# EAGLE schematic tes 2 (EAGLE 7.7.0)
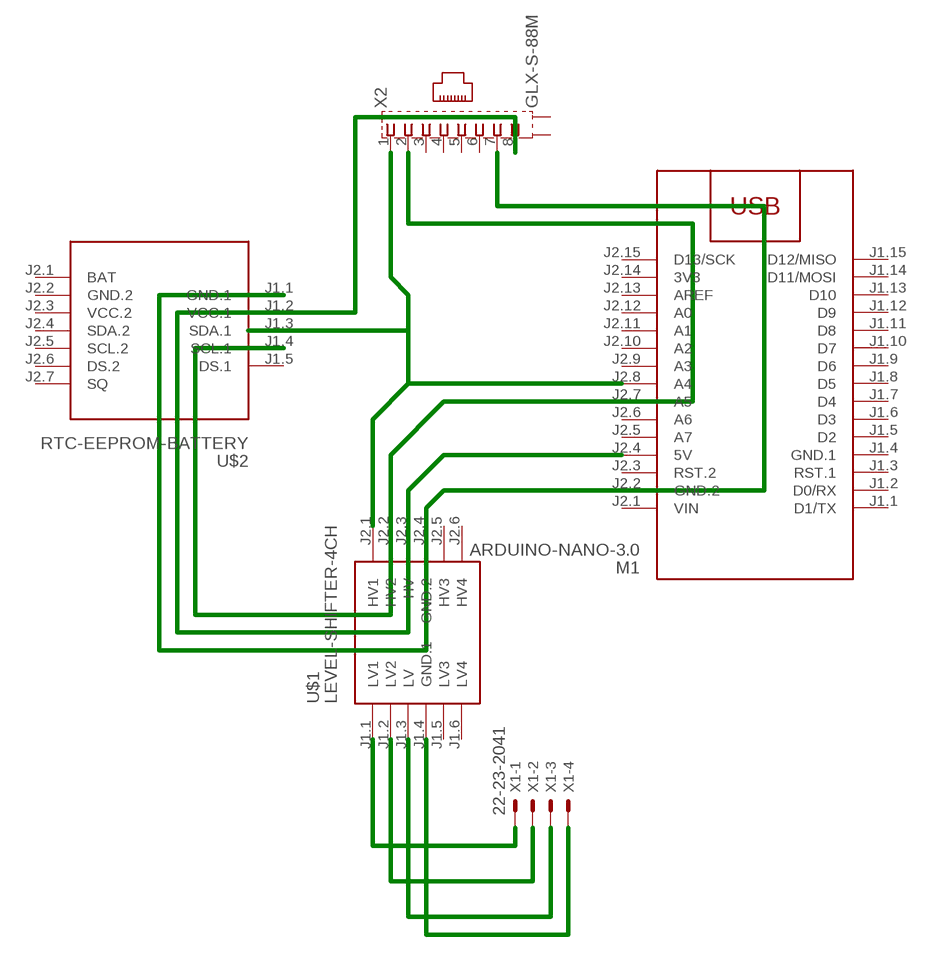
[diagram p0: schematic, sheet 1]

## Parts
M1  ARDUINO-NANO-3.0  [ARDUINO-NANO-3.0]
U$1  LEVEL-SHIFTER-4CH  [LEVEL-SHIFTER-4CH]
U$2  RTC-EEPROM-BATTERY  [RTC-EEPROM-BATTERY]
X1  22-23-2041  [22-23-2041]
X2  GLX-S-88M  [GLX-S-88M]

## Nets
N$1: M1.J2.2(GND.2) U$1.J2.4(GND.2) U$2.J1.1(GND.1) X2.7
N$2: M1.J2.4(5V) U$1.J2.3(HV) U$2.J1.2(VCC.1) X2.8
N$4: M1.J2.8(A4) U$1.J2.1(HV1) X2.1
N$5: U$1.J1.1(LV1) X1.1
N$6: U$1.J1.2(LV2) X1.2
N$7: U$1.J1.3(LV) X1.3
N$8: U$1.J1.4(GND.1) X1.4
N$9: M1.J2.7(A5) U$1.J2.2(HV2) U$2.J1.4(SCL.1) X2.2
Unconnected: M1.J1.1(D1/TX) M1.J1.2(D0/RX) M1.J1.3(RST.1) M1.J1.5(D2) M1.J1.6(D3) M1.J1.7(D4) M1.J1.8(D5) M1.J1.9(D6) M1.J1.10(D7) M1.J1.11(D8) M1.J1.12(D9) M1.J1.13(D10) M1.J1.14(D11/MOSI) M1.J1.15(D12/MISO) M1.J2.3(RST.2) M1.J2.5(A7) M1.J2.6(A6) M1.J2.9(A3) M1.J2.10(A2) M1.J2.11(A1) M1.J2.12(A0) M1.J2.13(AREF) M1.J2.15(D13/SCK) U$1.J1.5(LV3) U$1.J1.6(LV4) U$1.J2.5(HV3) U$1.J2.6(HV4) U$2.J1.3(SDA.1) U$2.J1.5(DS.1) U$2.J2.1(BAT) U$2.J2.4(SDA.2) U$2.J2.5(SCL.2) U$2.J2.6(DS.2) U$2.J2.7(SQ) X2.3 X2.4 X2.5 X2.6 X2.S1 X2.S2

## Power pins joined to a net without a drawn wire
3V3: M1.J2.14(3V3)
GND.1: M1.J1.4(GND.1)
GND.2: U$2.J2.2(GND.2)
VCC.2: U$2.J2.3(VCC.2)
VIN: M1.J2.1(VIN)

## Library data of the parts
M1 = diy-modules:ARDUINO-NANO-3.0: Arduino Nano 3.0 and compatible devices More details available here: https://www.arduino.cc/en/Main/ArduinoBoardNano Click here to find device on ebay.com
U$1 = diy-modules:LEVEL-SHIFTER-4CH: 4-Channel Bi-Directional Logic Level Converter based on BSS128 transistors Click here to find device on ebay.com
U$2 = diy-modules:RTC-EEPROM-BATTERY: RTC Module with Battery and EEPROM based on DS1307 and AT24C32 chips More details available here: http://henrysbench.capnfatz.com/henrys-bench/arduino-sensors-and-input/arduino-tiny-rtc-d1307-tutorial/ Click here to find device on ebay.com
X1 = con-molex:22-23-2041: .100" (2.54mm) Center Header - 4 Pin; MF: MOLEX; MPN: 22-23-2041; OC_FARNELL: 1462920; OC_NEWARK: 38C0355
X2 = con-kycon:GLX-S-88M: Mod. Jack, Right Angle, 8 posiotion, 8 contatcs RJ45 Source: GLX-S-88M.pdf; OC_FARNELL: unknown; OC_NEWARK: unknown

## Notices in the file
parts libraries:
diy-modules: Released under the Creative Commons Attribution 4.0 International License: http://creativecommons.org/licenses/by/4.0
